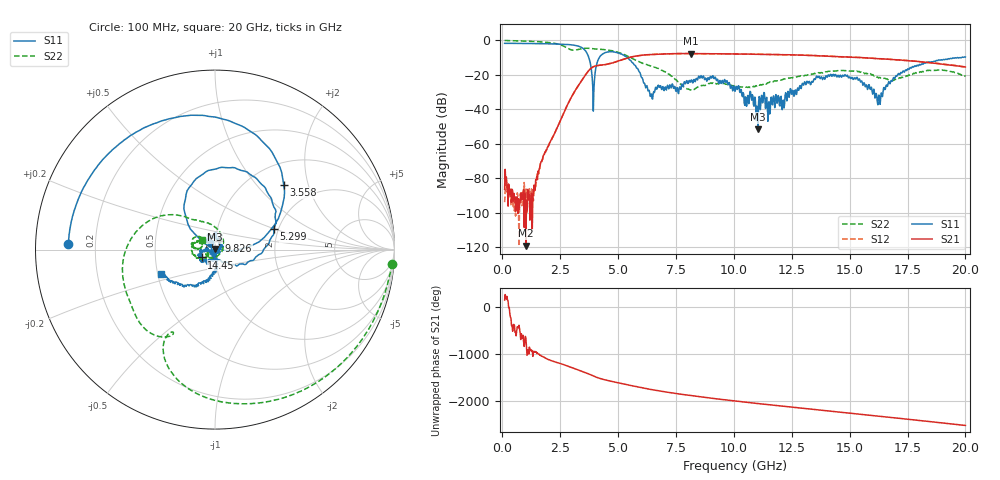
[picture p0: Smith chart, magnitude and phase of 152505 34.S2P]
!  2-Port S-parameters saved by WinCal
! VAR MeasName=S-Parameters (CALIBRATED_DATA) read from VNA (N5230C)
! VAR MeasDate=4/10/2015 9:31:51 AM
! VAR NAME=152505 34
! VAR FILENAME=152505 34.S2P
! VAR DATE=4/10/2015 9:31:51 AM
! VAR PHYS_PORTS=1,2
# Hz S DB R 50
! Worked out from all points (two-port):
!   801 points, 100 MHz to 20 GHz, reference 50 ohm
!   highest |S21| = -7.66 dB at 8.159 GHz (marker M1); lowest = -119.1 dB at 1.02 GHz (marker M2)
!   |S21| within 3 dB of the highest: 5.319 GHz to 16.22 GHz (10.9 GHz wide, 101 % of centre)
!   lowest |S11| = -51.7 dB at 11.04 GHz (marker M3), VSWR 1.01, Z = 49.9 + j0.213 ohm
!   |S11| at or under -10 dB: 3.735 GHz to 4.194 GHz (458.4 MHz wide, 11.6 % of centre); 5.388 GHz to 19.83 GHz (14.45 GHz wide, 115 % of centre)
!   |S22| runs from -29.0 to -0.1 dB; largest |S21 - S12| = 0.0056
!   S11 on the Smith chart (normalised r, x): 100 MHz: 0.10, +0.02; 3.558 GHz: 1.42, +1.41; 5.299 GHz: 1.89, +0.49; 9.826 GHz: 1.04, +0.10; 14.45 GHz: 0.86, -0.08; 20 GHz: 0.52, -0.16
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1e8  -1.75 177.6  -86.41 142.9  -93.92 -146.6  -0.08 -4.6
1.020375e9  -1.83 155.5  -119.13 41.0  -86.28 77.6  -0.46 -41.3
1.493e9  -1.91 143.5  -78.87 86.9  -78.71 82.0  -0.74 -60.8
2.562625e9  -2.24 109.8  -44.93 -136.1  -45.05 -136.7  -2.87 -110.3
3.43325e9  -4.23 57.4  -23.23 69.0  -23.24 69.3  -4.85 -121.8
3.557625e9  -5.59 43.2  -20.72 46.2  -20.73 46.4  -4.63 -126.9
3.93075e9  -41.07 60.3  -15.35 -32.5  -15.36 -32.2  -4.93 -143.3
4.32875e9  -7.97 106.9  -14.28 -100.4  -14.29 -100.7  -5.31 -159.0
5.298875e9  -9.20 19.0  -10.74 152.3  -10.73 152.5  -8.43 152.3
6.393375e9  -32.56 -148.8  -8.26 42.9  -8.27 43.0  -14.83 118.5
6.741625e9  -26.00 135.4  -8.03 13.6  -8.03 13.3  -16.36 103.9
8.1595e9  -23.09 127.7  -7.66 -90.1  -7.67 -90.2  -28.82 -48.6
9.826125e9  -25.58 65.3  -7.88 168.5  -7.87 168.4  -26.05 -154.2
1.005e10  -29.57 34.2  -7.90 155.6  -7.93 155.6  -26.67 -154.1
1.1045e10  -51.71 124.5  -8.10 101.4  -8.07 101.4  -25.79 -137.2
1.338325e10  -23.79 -111.5  -8.84 -21.2  -8.79 -21.0  -19.45 -152.9
1.445288e10  -21.29 -149.6  -9.45 -75.7  -9.44 -75.6  -17.66 -177.9
1.539812e10  -22.74 -177.5  -9.91 -123.2  -9.92 -123.7  -18.01 162.2
1.6219e10  -37.41 -131.6  -10.66 -165.6  -10.61 -165.1  -21.38 151.7
1.669162e10  -23.94 -80.6  -11.01 170.3  -10.99 169.9  -23.01 161.4
1.7811e10  -14.78 -103.7  -12.14 112.7  -12.07 112.0  -19.19 175.7
2e10  -9.70 -156.0  -15.50 -4.0  -15.48 -4.2  -21.02 144.0
